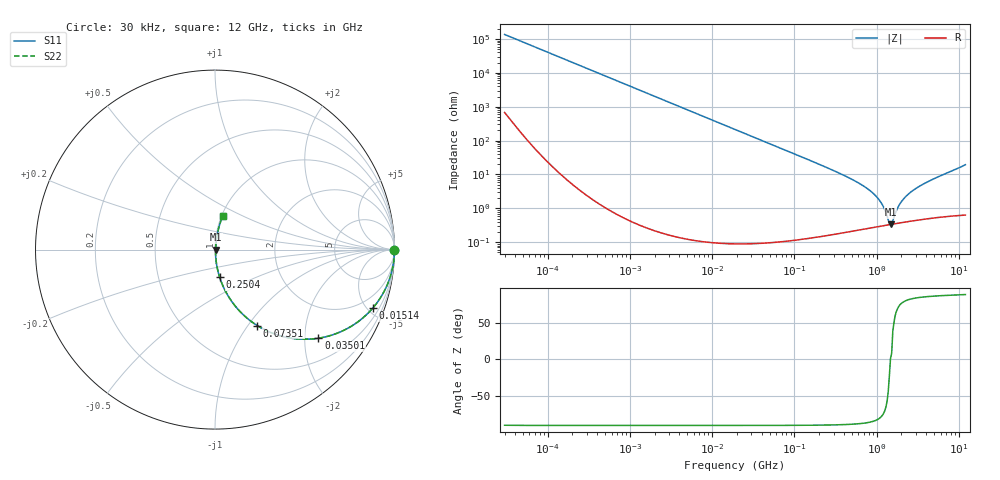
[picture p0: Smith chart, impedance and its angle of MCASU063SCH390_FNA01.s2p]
! MCASU063SCH390_FNA01  S-PARAMETER MODEL  ( General Type )
! Model Generated by TAIYO YUDEN Corporation (http://www.ty-top.com)
! Version 2.0
! TAIYO YUDEN Control No. 141022
! Copyright(c) 2013 TAIYO YUDEN CO.,LTD. All Rights Reserved.
! Product Description (link to TY-COMPAS)
! https://ds.yuden.co.jp/TYCOMPAS/or/detail?pn=MCASU063SCH390JFNA01&u=M
! Products Name : Multilayer Ceramic Capacitors
! Characteristics :
!  Capacitance : 39 pF , Rated Voltage : 50V , TCC : CH / C0H
!  Case Size : 0.6 x 0.3 / 0.024 x 0.012 [mm/inch] , Thickness : 0.3 / 0.012 [mm/inch]
!  (Conditions: Temperature = 25 degC , DC Bias Current/Voltage = 0A / 0V)
! External Node Assignments :
!  1  o---| |---o  2
! GND o---------o GND
! Frequency Range : 0.03MHz  -  12000MHz  [ 401 STEP ]
# MHz S RI R 50
! Freq[MHz].  S11 Real  S11 Imag  S21 Real  S21 Imag  S12 Real  S12 Imag  S22 Real  S22 Imag
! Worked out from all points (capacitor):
!   401 points, 30 kHz to 12 GHz, reference 50 ohm
!   read as one part in series: C = 39 pF near 32 kHz
!   lowest |Z| = 334 mohm at 1.475 GHz (marker M1)
!   series resonance near 1.473 GHz, so ESL is about 300 pH
!   S11 on the Smith chart (normalised r, x): 30 kHz: open; 15.14 MHz: 1.00, -5.39; 35.01 MHz: 1.00, -2.33; 73.51 MHz: 1.00, -1.11; 250.4 MHz: 1.00, -0.32; 12 GHz: 1.01, +0.39
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0.03  1 -0.000735  4.19e-06 0.000735  4.19e-06 0.000735  1 -0.000735
0.260295  1 -0.00638  4.19e-05 0.00638  4.19e-05 0.00638  1 -0.00638
2.258455  0.9969 -0.0552  0.00306 0.0552  0.00306 0.0552  0.9969 -0.0552
6.13721  0.9779 -0.1471  0.0221 0.1471  0.0221 0.1471  0.9779 -0.1471
15.13963  0.8789 -0.3261  0.1211 0.3261  0.1211 0.3261  0.8789 -0.3261
18.97367  0.8221 -0.3822  0.1779 0.3822  0.1779 0.3822  0.8221 -0.3822
35.01459  0.5756 -0.4939  0.4244 0.4939  0.4244 0.4939  0.5756 -0.4939
73.51358  0.2351 -0.4231  0.7649 0.4231  0.7649 0.4231  0.2351 -0.4231
164.6252  0.0576 -0.2303  0.9424 0.2303  0.9424 0.2303  0.0576 -0.2303
250.359  0.0259 -0.1539  0.9741 0.1539  0.9741 0.1539  0.0259 -0.1539
542.8588  0.00633 -0.0643  0.9937 0.0643  0.9937 0.0643  0.00633 -0.0643
880.5704  0.00354 -0.0294  0.9965 0.0294  0.9965 0.0294  0.00354 -0.0294
1139.739  0.00319 -0.014  0.9968 0.014  0.9968 0.014  0.00319 -0.014
1255.512  0.00319 -0.00855  0.9968 0.00855  0.9968 0.00855  0.00319 -0.00855
1428.372  0.00329 -0.00137  0.9967 0.00137  0.9967 0.00137  0.00329 -0.00137
1475.185  0.00333 7.32e-05  0.9967 -7.32e-05  0.9967 -7.32e-05  0.00333 7.32e-05
1573.464  0.00343 0.00269  0.9966 -0.00269  0.9966 -0.00269  0.00343 0.00269
1790.1  0.00369 0.00912  0.9963 -0.00912  0.9963 -0.00912  0.00369 0.00912
1971.936  0.00396 0.0145  0.996 -0.0145  0.996 -0.0145  0.00396 0.0145
2635.962  0.00511 0.0304  0.9949 -0.0304  0.9949 -0.0304  0.00511 0.0304
4415.924  0.00912 0.064  0.9909 -0.064  0.9909 -0.064  0.00912 0.064
12000  0.0421 0.1852  0.9579 -0.1852  0.9579 -0.1852  0.0421 0.1852
